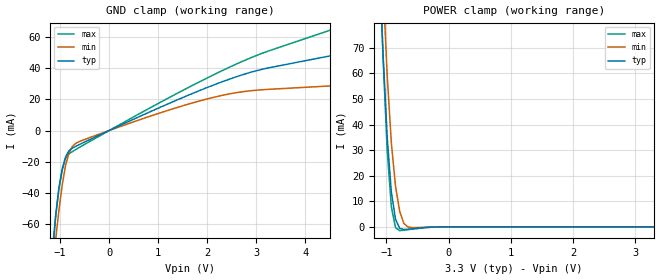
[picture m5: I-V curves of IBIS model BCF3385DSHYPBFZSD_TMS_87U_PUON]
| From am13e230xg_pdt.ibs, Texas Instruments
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|   Model BCF3385DSHYPBFZSD_TMS_87U_PUON
[Model] BCF3385DSHYPBFZSD_TMS_87U_PUON
Model_type Input
Polarity   Non-Inverting
Enable   Active-High
Vinl =  0.990V
Vinh =  2.310V
C_comp   0.563pF   0.511pF   0.622pF
[Model Spec]
Vinh   2.310V   2.079V   2.541V
Vinl   0.990V   0.891V   1.089V
[Temperature Range]   25.000   0.155k   -40.000
[Voltage Range]   3.300V   2.970V   3.630V
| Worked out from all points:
|   GND clamp passes 1 mA (typ) near -0.07 V on its own axis
|   POWER clamp passes 1 mA (typ) near -0.70 V on its own axis
[GND_clamp]
|Voltage   I(typ)   I(min)   I(max)
-3.3V     -1.011A    -885.1mA   -1.28A
-1.156V   -76.97mA   -90.47mA   -80.68mA
-1.089V   -54.44mA   -69.82mA   -54.87mA
-1.022V   -36.36mA   -50.92mA   -37.27mA
-955mV    -24.31mA   -34.72mA   -25.38mA
-888mV    -16.92mA   -22.46mA   -17.88mA
-821mV    -13.06mA   -14.65mA   -15.07mA
-754mV    -11.39mA   -10.44mA   -13.64mA
1.189V    17.02mA    12.89mA    20.64mA
2.328V    31.68mA    22.8mA     38.93mA
3.266V    40.45mA    26.55mA    51.4mA
6.6V      60.98mA    32.38mA    86.97mA
[POWER_clamp]
|Voltage   I(typ)   I(min)   I(max)
-3.3V     1.722A     1.973A     1.84A
-1.122V   107.3mA    137.2mA    110.6mA
-1.055V   67.75mA    94.81mA    66.49mA
-988mV    34.98mA    59.07mA    29.84mA
-921mV    13.5mA     32.68mA    7.837mA
-854mV    2.984mA    15.84mA    -313.8uA
-787mV    -613.5uA   5.993mA    -1.478mA
-720mV    -1.034mA   1.322mA    -1.323mA
-653mV    -912.6uA   -59.76uA   -1.106mA
-586mV    -746.5uA   -298.4uA   -897.7uA
-117mV    0A         0A         0A
3.3V      0A         0A         0A
